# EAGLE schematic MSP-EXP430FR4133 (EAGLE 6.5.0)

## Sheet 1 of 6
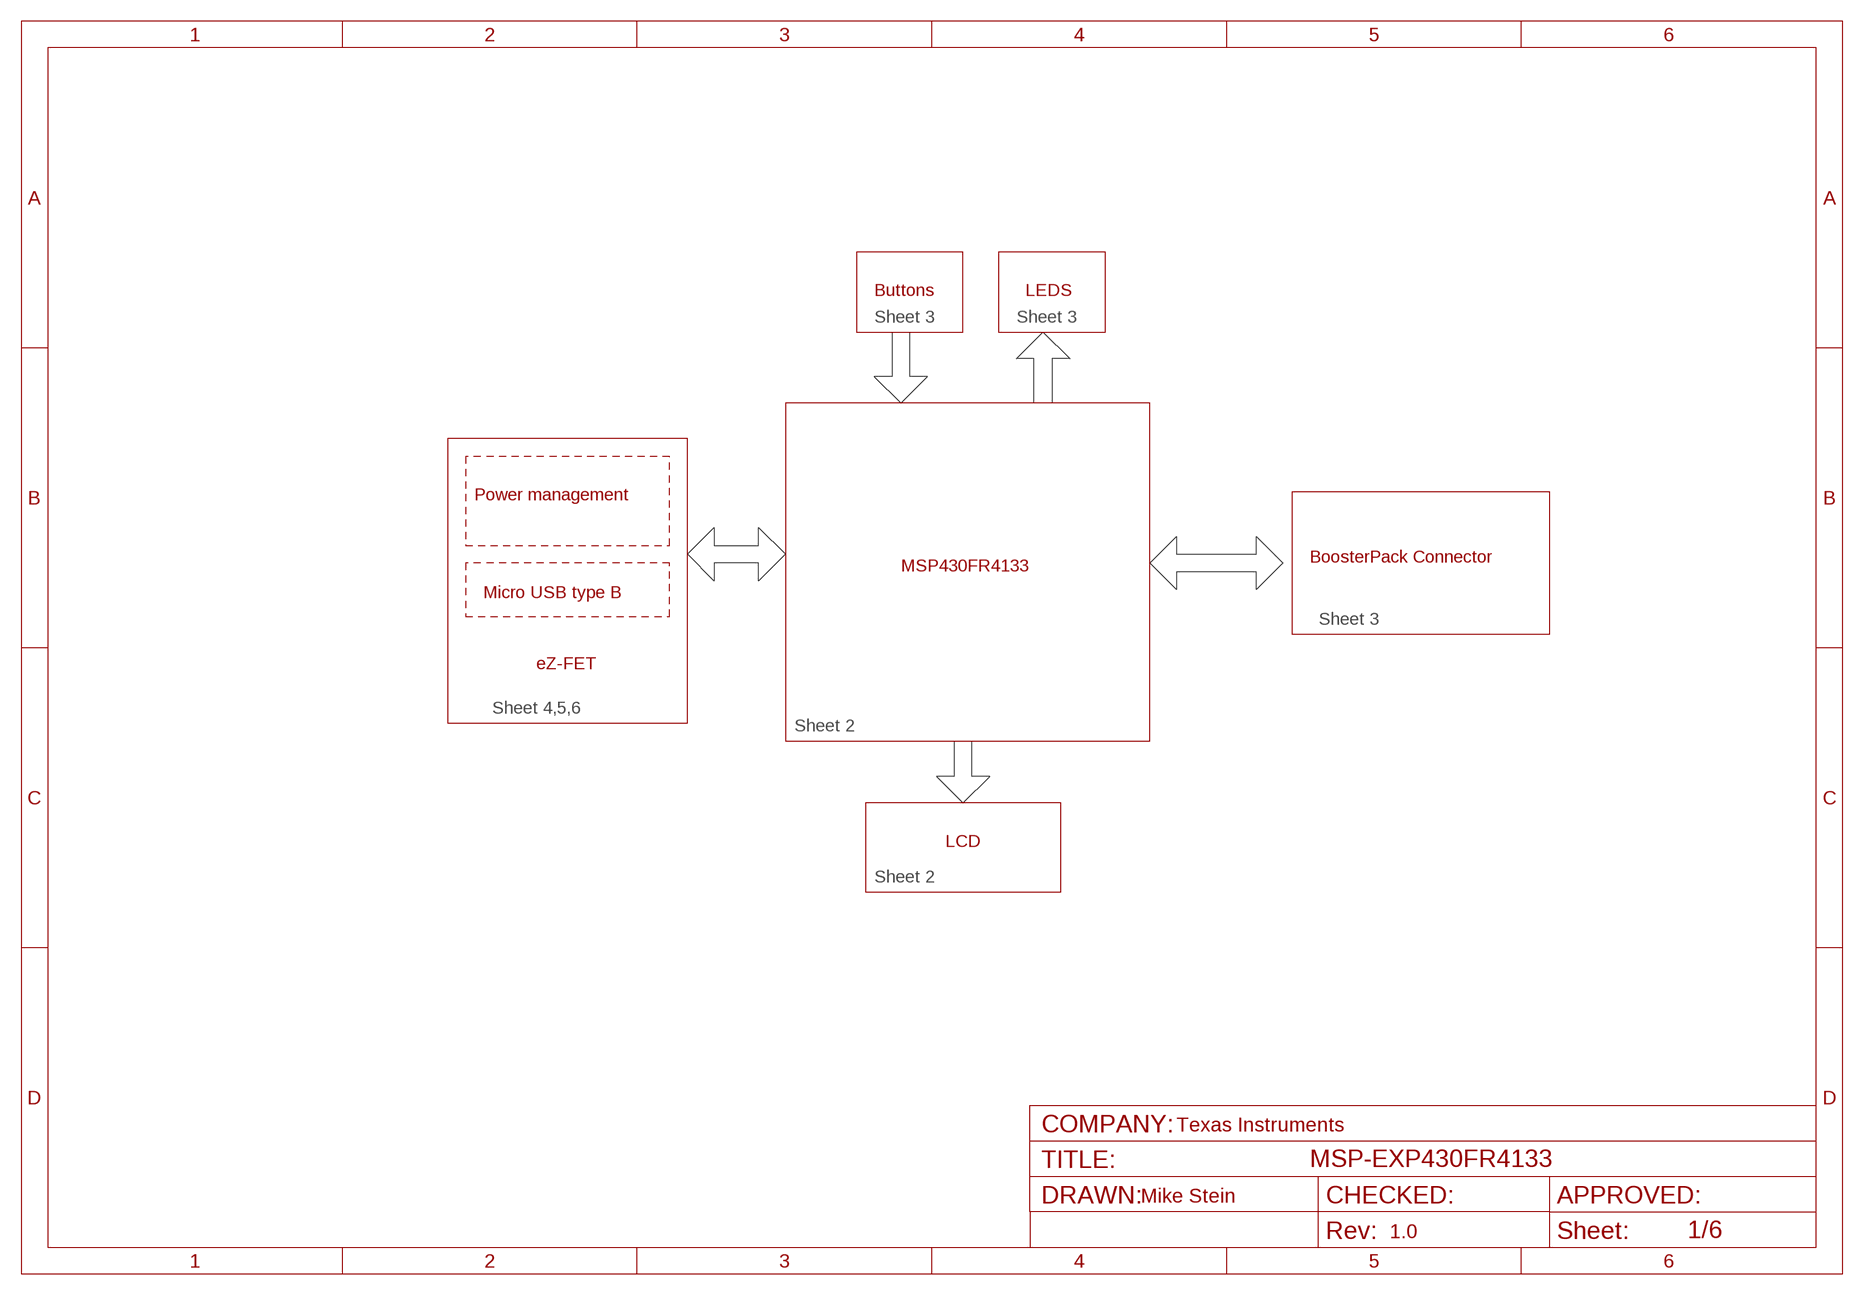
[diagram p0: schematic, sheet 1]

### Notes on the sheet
- Buttons | LEDS
- Sheet 3 | Sheet 3
- Power management
- BoosterPack Connector
- MSP430FR4133
- Micro USB type B
- Sheet 3
- eZ-FET
- Sheet 4,5,6
- Sheet 2
- LCD
- Sheet 2
- Texas Instruments
- Mike Stein
- 1.0

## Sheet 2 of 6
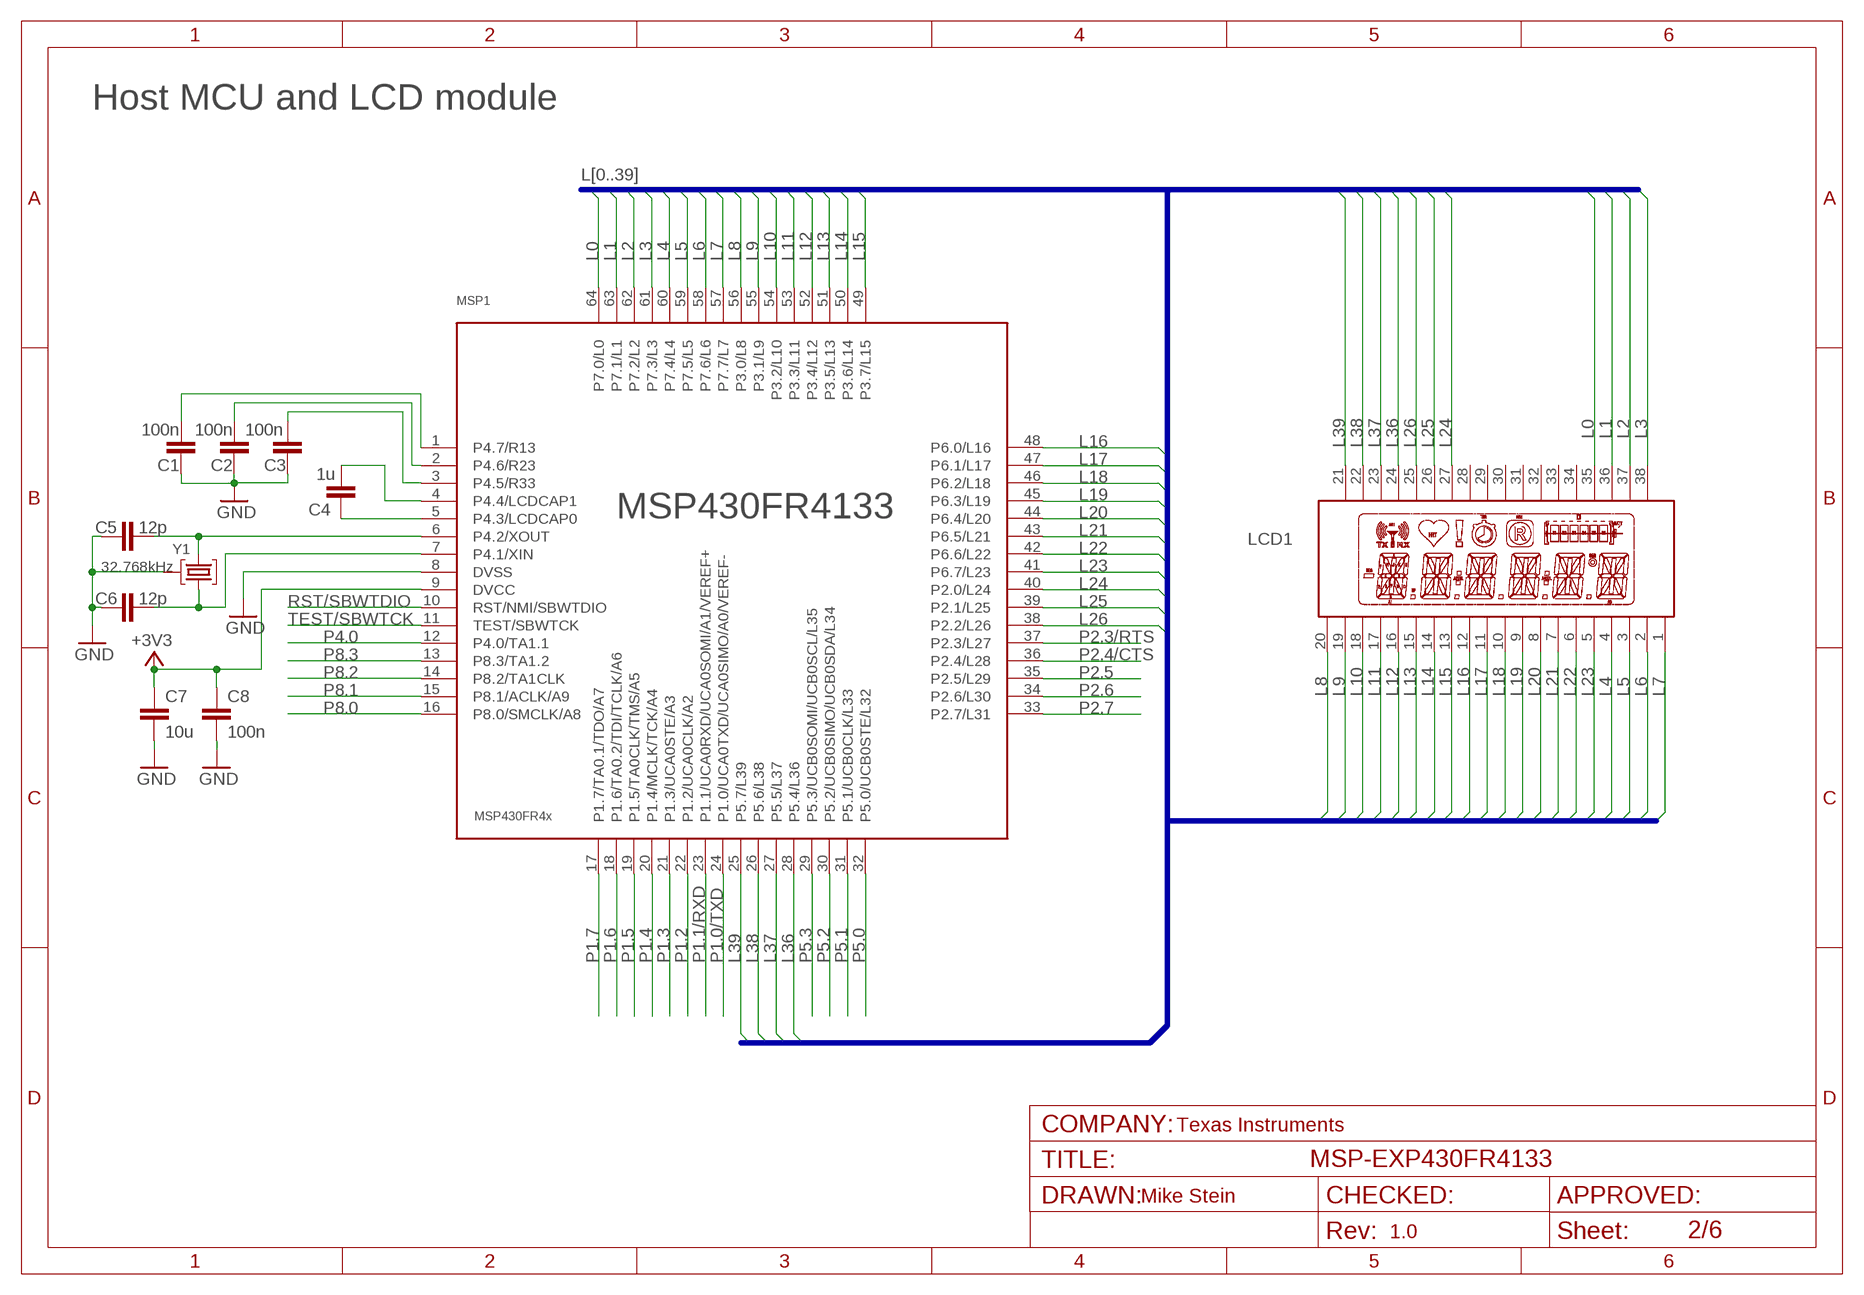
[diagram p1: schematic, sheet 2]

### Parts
C1  100n  C-EUC0402  [C0402]
C2  100n  C-EUC0402  [C0402]
C3  100n  C-EUC0402  [C0402]
C4  1u  C-EUC0402  [C0402]
C5  12p  C-EUC0402  [C0402]
C6  12p  C-EUC0402  [C0402]
C7  10u  C-EUC0603  [C0603]
C8  100n  C-EUC0402  [C0402]
LCD1  FH1138P  [FH1138P]
MSP1  MSP430FR4x  MSP430G621IPM  [LQFP64]
Y1  32.768kHz  MS3V-T1R  [MS3V-T1R]

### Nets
+3V3: C7.1 C8.1 MSP1.9(DVCC) ; also sheet 3,5
GND: C1.2 C2.2 C3.2 C5.2 C6.2 C7.2 C8.2 MSP1.8(DVSS) Y1.P3(GND) ; also sheet 3,4,5,6
L0: LCD1.35 MSP1.64(P7.0/L0)
L1: LCD1.36 MSP1.63(P7.1/L1)
L2: LCD1.37 MSP1.62(P7.2/L2)
L3: LCD1.38 MSP1.61(P7.3/L3)
L4: LCD1.4 MSP1.60(P7.4/L4)
L5: LCD1.3 MSP1.59(P7.5/L5)
L6: LCD1.2 MSP1.58(P7.6/L6)
L7: LCD1.1 MSP1.57(P7.7/L7)
L8: LCD1.20 MSP1.56(P3.0/L8)
L9: LCD1.19 MSP1.55(P3.1/L9)
L10: LCD1.18 MSP1.54(P3.2/L10)
L11: LCD1.17 MSP1.53(P3.3/L11)
L12: LCD1.16 MSP1.52(P3.4/L12)
L13: LCD1.15 MSP1.51(P3.5/L13)
L14: LCD1.14 MSP1.50(P3.6/L14)
L15: LCD1.13 MSP1.49(P3.7/L15)
L16: LCD1.12 MSP1.48(P6.0/L16)
L17: LCD1.11 MSP1.47(P6.1/L17)
L18: LCD1.10 MSP1.46(P6.2/L18)
L19: LCD1.9 MSP1.45(P6.3/L19)
L20: LCD1.8 MSP1.44(P6.4/L20)
L21: LCD1.7 MSP1.43(P6.5/L21)
L22: LCD1.6 MSP1.42(P6.6/L22)
L23: LCD1.5 MSP1.41(P6.7/L23)
L24: LCD1.27 MSP1.40(P2.0/L24)
L25: LCD1.26 MSP1.39(P2.1/L25)
L26: LCD1.25 MSP1.38(P2.2/L26)
L36: LCD1.24 MSP1.28(P5.4/L36)
L37: LCD1.23 MSP1.27(P5.5/L37)
L38: LCD1.22 MSP1.26(P5.6/L38)
L39: LCD1.21 MSP1.25(P5.7/L39)
N$4: C1.1 MSP1.1(P4.7/R13)
N$10: C2.1 MSP1.2(P4.6/R23)
N$11: C4.1 MSP1.4(P4.4/LCDCAP1)
N$14: C5.1 MSP1.6(P4.2/XOUT) Y1.P2
N$17: C4.2 MSP1.5(P4.3/LCDCAP0)
N$18: C6.1 MSP1.7(P4.1/XIN) Y1.P1
N$19: C3.1 MSP1.3(P4.5/R33)
P1.0/TXD: MSP1.24(P1.0/UCA0TXD/UCA0SIMO/A0/VEREF-) ; also sheet 3,5
P1.1/RXD: MSP1.23(P1.1/UCA0RXD/UCA0SOMI/A1/VEREF+) ; also sheet 3,5
P1.2: MSP1.22(P1.2/UCA0CLK/A2) ; also sheet 3
P1.3: MSP1.21(P1.3/UCA0STE/A3) ; also sheet 3
P1.4: MSP1.20(P1.4/MCLK/TCK/A4) ; also sheet 3
P1.5: MSP1.19(P1.5/TA0CLK/TMS/A5) ; also sheet 3
P1.6: MSP1.18(P1.6/TA0.2/TDI/TCLK/A6) ; also sheet 3
P1.7: MSP1.17(P1.7/TA0.1/TDO/A7) ; also sheet 3
P2.3/RTS: MSP1.37(P2.3/L27) ; also sheet 5
P2.4/CTS: MSP1.36(P2.4/L28) ; also sheet 5
P2.5: MSP1.35(P2.5/L29) ; also sheet 3
P2.6: MSP1.34(P2.6/L30) ; also sheet 3
P2.7: MSP1.33(P2.7/L31) ; also sheet 3
P4.0: MSP1.12(P4.0/TA1.1) ; also sheet 3
P5.0: MSP1.32(P5.0/UCB0STE/L32) ; also sheet 3
P5.1: MSP1.31(P5.1/UCB0CLK/L33) ; also sheet 3
P5.2: MSP1.30(P5.2/UCB0SIMO/UCB0SDA/L34) ; also sheet 3
P5.3: MSP1.29(P5.3/UCB0SOMI/UCB0SCL/L35) ; also sheet 3
P8.0: MSP1.16(P8.0/SMCLK/A8) ; also sheet 3
P8.1: MSP1.15(P8.1/ACLK/A9) ; also sheet 3
P8.2: MSP1.14(P8.2/TA1CLK) ; also sheet 3
P8.3: MSP1.13(P8.3/TA1.2) ; also sheet 3
RST/SBWTDIO: MSP1.10(RST/NMI/SBWTDIO) ; also sheet 3,5
TEST/SBWTCK: MSP1.11(TEST/SBWTCK) ; also sheet 5
Unconnected: LCD1.28 LCD1.29 LCD1.30 LCD1.31 LCD1.32 LCD1.33 LCD1.34

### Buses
L[0..39]

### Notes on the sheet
- Host MCU and LCD module
- MSP430FR4133
- Texas Instruments
- Mike Stein
- 1.0

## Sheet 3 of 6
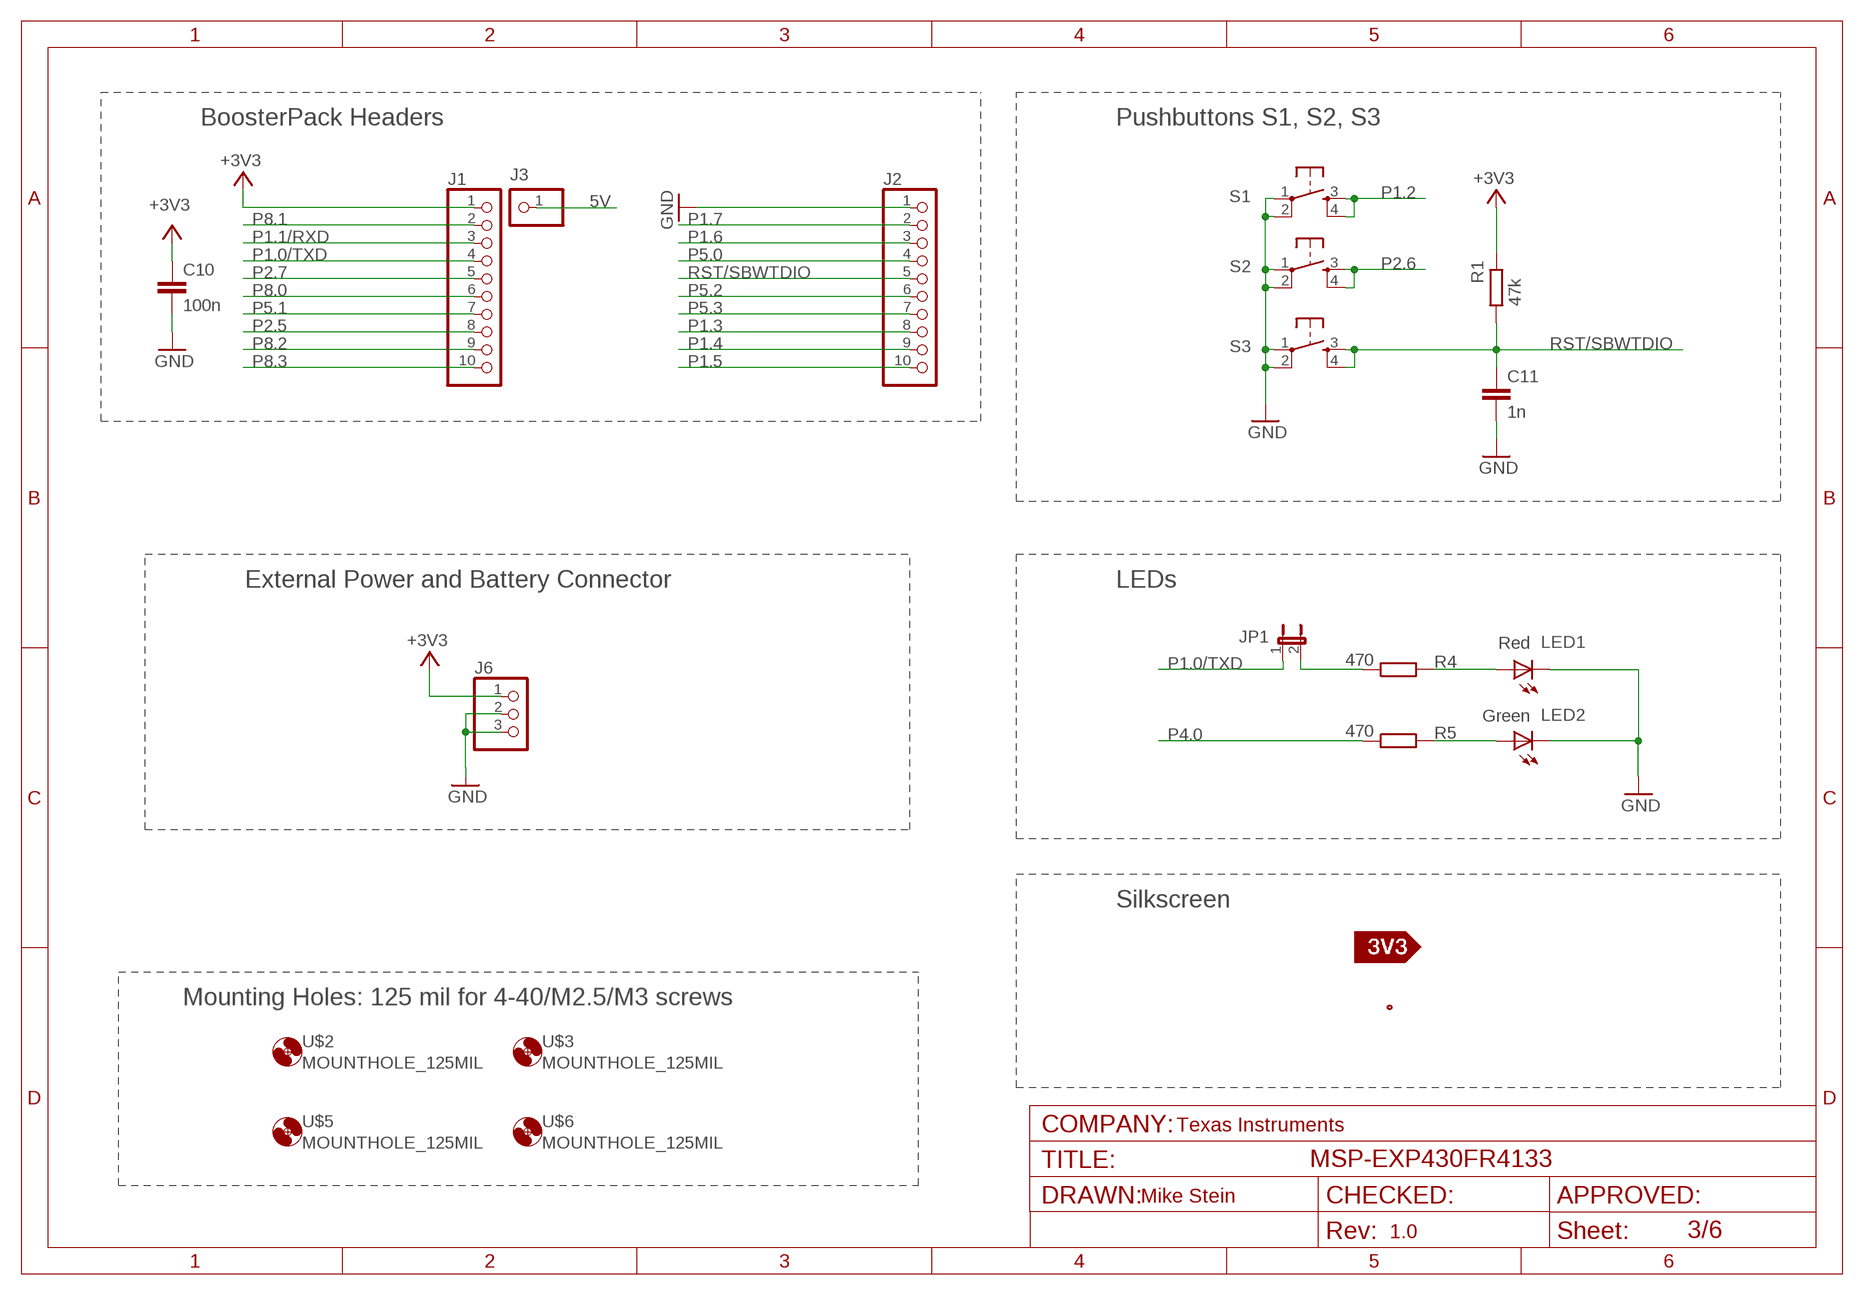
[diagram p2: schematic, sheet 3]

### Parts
C10  100n  C-EUC0402  [C0402]
C11  1n  C-EUC0402  [C0402]
J1  PINHEADER1X10  [PINHEAFER1X10]
J2  PINHEADER1X10  [PINHEAFER1X10]
J3  TEST_PIN2  PINHD-1X1  [1X01]
J6  PINHEADER1X3  [PINHEADER1X3]
JP1  JUMPER_2.51MM  [JUMPER-2.54]
LED1  Red  CHIP-LED  [LED0805]
LED2  Green  CHIP-LED  [LED0805]
R1  47k  R-EU_  [R0402]
R4  470  R-EU_  [R0402]
R5  470  R-EU_  [R0402]
S1  T062S  [T062S]
S2  T062S  [T062S]
S3  T062S  [T062S]
U$2  MOUNTHOLE_125MIL  [MOUNTHOLE_125MIL]
U$3  MOUNTHOLE_125MIL  [MOUNTHOLE_125MIL]
U$5  MOUNTHOLE_125MIL  [MOUNTHOLE_125MIL]
U$6  MOUNTHOLE_125MIL  [MOUNTHOLE_125MIL]
U$7  SILK_3V3_TAG  [SILK_3V3_TAG]
U$8  SILK_FR4133_REAR_REV02  [SILK_FR4133_REAR_REV02]

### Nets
5V: J3.1 ; also sheet 5
+3V3: C10.1 J1.1 J6.1 R1.1 ; also sheet 2,5
GND: C10.2 C11.2 J2.1 J6.2 J6.3 LED1.C LED2.C S1.1 S1.2 S2.1 S2.2 S3.1 S3.2 ; also sheet 2,4,5,6
N$6: JP1.2 R4.1
N$7: LED1.A R4.2
N$8: LED2.A R5.2
P1.0/TXD: J1.4 JP1.1 ; also sheet 2,5
P1.1/RXD: J1.3 ; also sheet 2,5
P1.2: S1.3 S1.4 ; also sheet 2
P1.3: J2.8 ; also sheet 2
P1.4: J2.9 ; also sheet 2
P1.5: J2.10 ; also sheet 2
P1.6: J2.3 ; also sheet 2
P1.7: J2.2 ; also sheet 2
P2.5: J1.8 ; also sheet 2
P2.6: S2.3 S2.4 ; also sheet 2
P2.7: J1.5 ; also sheet 2
P4.0: R5.1 ; also sheet 2
P5.0: J2.4 ; also sheet 2
P5.1: J1.7 ; also sheet 2
P5.2: J2.6 ; also sheet 2
P5.3: J2.7 ; also sheet 2
P8.0: J1.6 ; also sheet 2
P8.1: J1.2 ; also sheet 2
P8.2: J1.9 ; also sheet 2
P8.3: J1.10 ; also sheet 2
RST/SBWTDIO: C11.1 J2.5 R1.2 S3.3 S3.4 ; also sheet 2,5

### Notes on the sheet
- BoosterPack Headers | Pushbuttons S1, S2, S3
- External Power and Battery Connector | LEDs
- Silkscreen
- Mounting Holes: 125 mil for 4-40/M2.5/M3 screws
- Texas Instruments
- Mike Stein
- 1.0

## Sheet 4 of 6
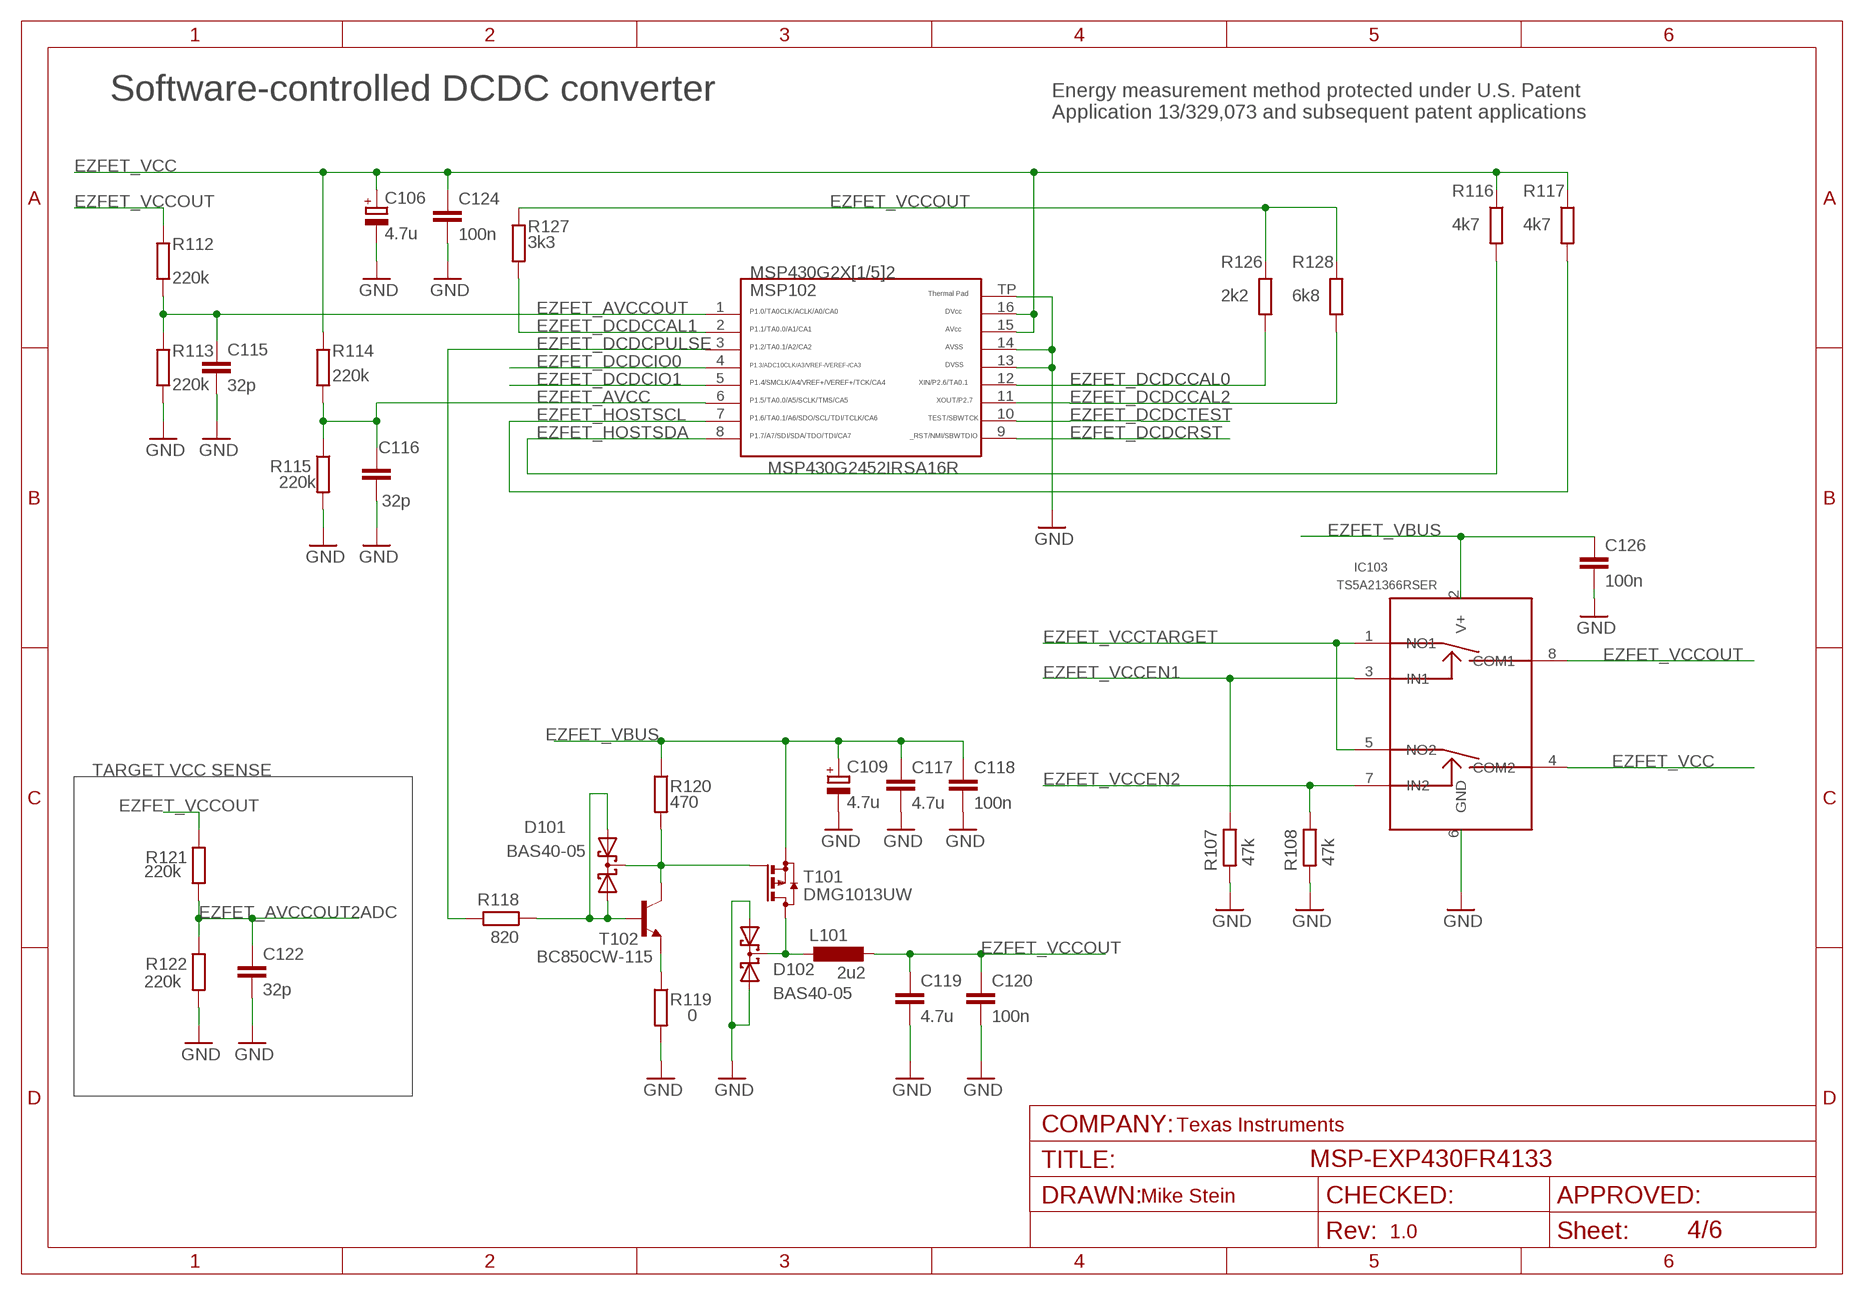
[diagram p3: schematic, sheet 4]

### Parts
C106  4.7u  CPOL-EUA/3216-18R  [A/3216-18R]
C109  4.7u  CPOL-EUA/3216-18R  [A/3216-18R]
C115  32p  C-EUC0402  [C0402]
C116  32p  C-EUC0402  [C0402]
C117  4.7u  C-EUC0603  [C0603]
C118  100n  C-EUC0402  [C0402]
C119  4.7u  C-EUC0603  [C0603]
C120  100n  C-EUC0402  [C0402]
C122  32p  C-EUC0402  [C0402]
C124  100n  C-EUC0402  [C0402]
C126  100n  C-EUC0402  [C0402]
D101  BAS40-05  BAS40-05W  [SOT323]
D102  BAS40-05  BAS40-05W  [SOT323]
IC103  TS5A21366RSER  [UQFN_RSE]
L101  2u2  L-EUL3216C  [L3216C]
MSP102  MSP430G2452IRSA16R  G2X[1/5]2---RSA16  [RSA16]
R107  47k  R-EU_  [R0402]
R108  47k  R-EU_  [R0402]
R112  220k  R-EU_  [R0402]
R113  220k  R-EU_  [R0402]
R114  220k  R-EU_  [R0402]
R115  220k  R-EU_  [R0402]
R116  4k7  R-EU_  [R0402]
R117  4k7  R-EU_  [R0402]
R118  820  R-EU_  [R0402]
R119  0  R-EU_  [R0402]
R120  470  R-EU_  [R0402]
R121  220k  R-EU_  [R0402]
R122  220k  R-EU_  [R0402]
R126  2k2  R-EU_  [R0402]
R127  3k3  R-EU_  [R0402]
R128  6k8  R-EU_  [R0402]
T101  DMG1013UW  [SOT323]
T102  BC850CW-115  [SOT323]

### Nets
EZFET_AVCC: C116.2 MSP102.6 R114.2 R115.1
EZFET_AVCCOUT: C115.2 MSP102.1 R112.2 R113.1
EZFET_AVCCOUT2ADC: C122.2 R121.2 R122.1 ; also sheet 5
EZFET_DCDCCAL0: MSP102.12 R126.2
EZFET_DCDCCAL1: MSP102.2 R127.2
EZFET_DCDCCAL2: MSP102.11 R128.2
EZFET_DCDCIO0: MSP102.4 ; also sheet 5
EZFET_DCDCIO1: MSP102.5 ; also sheet 5
EZFET_DCDCPULSE: MSP102.3 R118.2 ; also sheet 5
EZFET_DCDCRST: MSP102.9 ; also sheet 5,6
EZFET_DCDCTEST: MSP102.10 ; also sheet 5,6
EZFET_HOSTSCL: MSP102.7 R117.2 ; also sheet 5
EZFET_HOSTSDA: MSP102.8 R116.2 ; also sheet 5
EZFET_VBUS: C109.+ C117.1 C118.1 C126.1 IC103.2(V+) R120.1 T101.2(S) ; also sheet 5,6
EZFET_VCC: C106.+ C124.1 IC103.4(COM2) MSP102.15 MSP102.16 R114.1 R116.1 R117.1 ; also sheet 5,6
EZFET_VCCEN1: IC103.3(IN1) R107.1 ; also sheet 5
EZFET_VCCEN2: IC103.7(IN2) R108.1 ; also sheet 5
EZFET_VCCOUT: C119.1 C120.1 IC103.8(COM1) L101.2 R112.1 R121.1 R126.1 R127.1 R128.1
EZFET_VCCTARGET: IC103.1(NO1) IC103.5(NO2) ; also sheet 5
GND: C106.- C109.- C115.1 C116.1 C117.2 C118.2 C119.2 C120.2 C122.1 C124.2 C126.2 D102.1(A1) D102.2(A2) IC103.6(GND) MSP102.13 MSP102.14 MSP102.TP R107.2 R108.2 R113.2 R115.2 R119.2 R122.2 ; also sheet 2,3,5,6
N$12: R119.1 T102.2(E)
N$13: D101.1(A1) D101.2(A2) R118.1 T102.1(B)
N$15: D102.3(C) L101.1 T101.3(D)
N$16: D101.3(C) R120.2 T101.1(G) T102.3(C)

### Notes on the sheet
- Software-controlled DCDC converter
- Energy measurement method protected under U.S. Patent 
  Application 13/329,073 and subsequent patent applications
- MSP430G2452IRSA16R
- TARGET VCC SENSE
- Texas Instruments
- Mike Stein
- 1.0

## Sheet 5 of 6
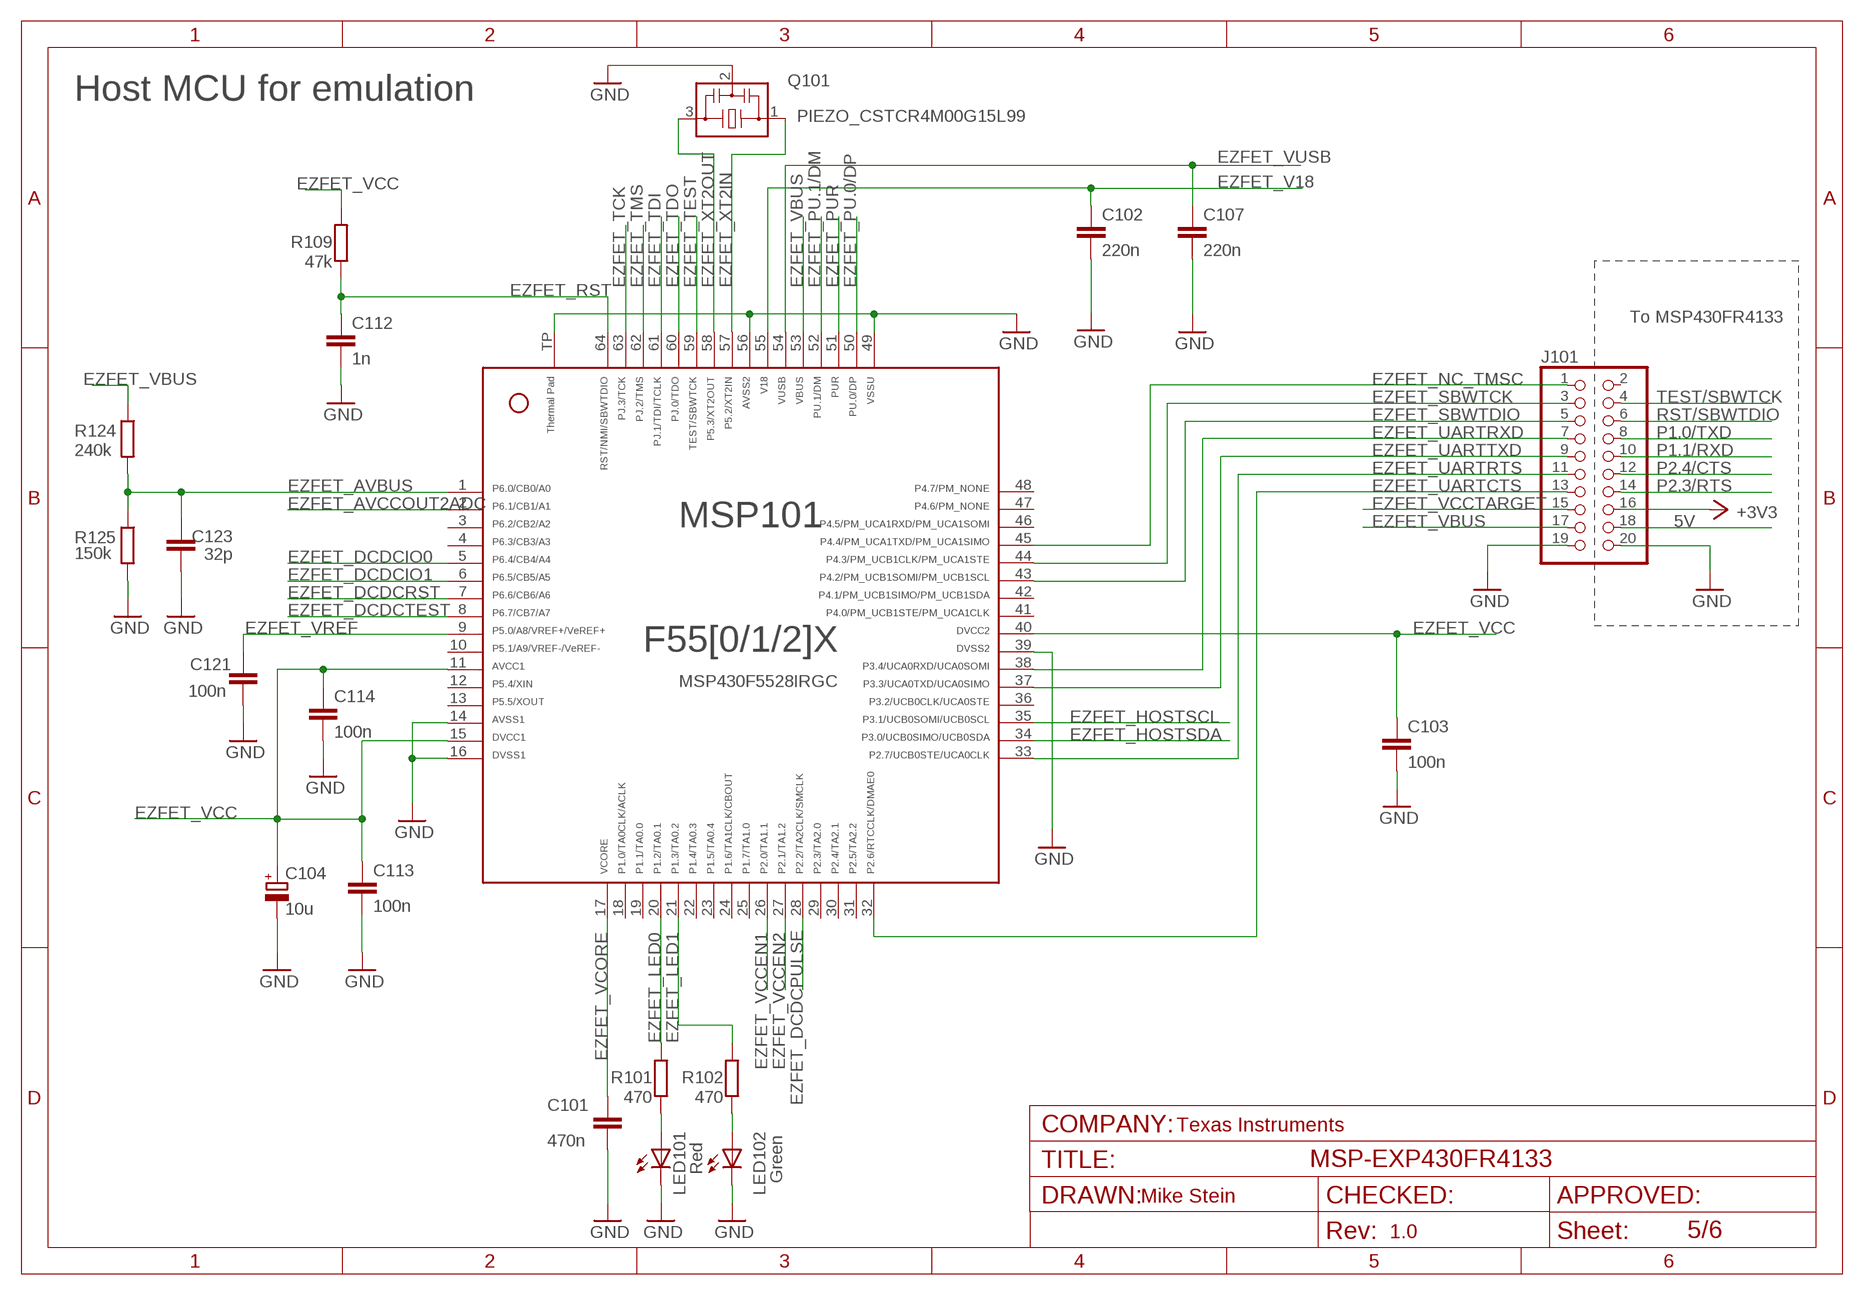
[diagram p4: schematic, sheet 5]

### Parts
C101  470n  C-EUC0402  [C0402]
C102  220n  C-EUC0402  [C0402]
C103  100n  C-EUC0402  [C0402]
C104  10u  CPOL-EUA/3216-18R  [A/3216-18R]
C107  220n  C-EUC0402  [C0402]
C112  1n  C-EUC0402  [C0402]
C113  100n  C-EUC0402  [C0402]
C114  100n  C-EUC0402  [C0402]
C121  100n  C-EUC0402  [C0402]
C123  32p  C-EUC0402  [C0402]
J101  PINHD-2X10  [2X10]
LED101  Red  CHIP-LED  [LED0805]
LED102  Green  CHIP-LED  [LED0805]
MSP101  MSP430F5528IRGC  F55[0/1/2]X---RGC64  [RGC64]
Q101  PIEZO_CSTCR4M00G15L99  CSTCR4M  [CSTCR4M]
R101  470  R-EU_  [R0402]
R102  470  R-EU_  [R0402]
R109  47k  R-EU_  [R0402]
R124  240k  R-EU_  [R0402]
R125  150k  R-EU_  [R0402]

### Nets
5V: J101.18 ; also sheet 3
+3V3: J101.16 ; also sheet 2,3
EZFET_AVBUS: C123.2 MSP101.1 R124.2 R125.1
EZFET_AVCCOUT2ADC: MSP101.2 ; also sheet 4
EZFET_DCDCIO0: MSP101.5 ; also sheet 4
EZFET_DCDCIO1: MSP101.6 ; also sheet 4
EZFET_DCDCPULSE: MSP101.28 ; also sheet 4
EZFET_DCDCRST: MSP101.7 ; also sheet 4,6
EZFET_DCDCTEST: MSP101.8 ; also sheet 4,6
EZFET_HOSTSCL: MSP101.35 ; also sheet 4
EZFET_HOSTSDA: MSP101.34 ; also sheet 4
EZFET_LED0: MSP101.20 R101.2
EZFET_LED1: MSP101.21 R102.2
EZFET_NC_TMSC: J101.1 MSP101.45
EZFET_PU.0/DP: MSP101.50 ; also sheet 6
EZFET_PU.1/DM: MSP101.52 ; also sheet 6
EZFET_PUR: MSP101.51 ; also sheet 6
EZFET_RST: C112.1 MSP101.64 R109.1 ; also sheet 6
EZFET_SBWTCK: J101.3 MSP101.44
EZFET_SBWTDIO: J101.5 MSP101.43
EZFET_TCK: MSP101.63 ; also sheet 6
EZFET_TDI: MSP101.61 ; also sheet 6
EZFET_TDO: MSP101.60 ; also sheet 6
EZFET_TEST: MSP101.59 ; also sheet 6
EZFET_TMS: MSP101.62 ; also sheet 6
EZFET_UARTCTS: J101.13 MSP101.32
EZFET_UARTRTS: J101.11 MSP101.33
EZFET_UARTRXD: J101.7 MSP101.38
EZFET_UARTTXD: J101.9 MSP101.37
EZFET_V18: C102.1 MSP101.55
EZFET_VBUS: J101.17 MSP101.53 R124.1 ; also sheet 4,6
EZFET_VCC: C103.1 C104.+ C113.1 C114.1 MSP101.11 MSP101.15 MSP101.40 R109.2 ; also sheet 4,6
EZFET_VCCEN1: MSP101.26 ; also sheet 4
EZFET_VCCEN2: MSP101.27 ; also sheet 4
EZFET_VCCTARGET: J101.15 ; also sheet 4
EZFET_VCORE: C101.1 MSP101.17
EZFET_VREF: C121.1 MSP101.9
EZFET_VUSB: C107.1 MSP101.54
EZFET_XT2IN: MSP101.57 Q101.1
EZFET_XT2OUT: MSP101.58 Q101.3
GND: C101.2 C102.2 C103.2 C104.- C107.2 C112.2 C113.2 C114.2 C121.2 C123.1 J101.19 J101.20 LED101.C LED102.C MSP101.14 MSP101.16 MSP101.39 MSP101.49 MSP101.56 MSP101.TP Q101.2 R125.2 ; also sheet 2,3,4,6
N$1: LED101.A R101.1
N$2: LED102.A R102.1
P1.0/TXD: J101.8 ; also sheet 2,3
P1.1/RXD: J101.10 ; also sheet 2,3
P2.3/RTS: J101.14 ; also sheet 2
P2.4/CTS: J101.12 ; also sheet 2
RST/SBWTDIO: J101.6 ; also sheet 2,3
TEST/SBWTCK: J101.4 ; also sheet 2
Unconnected: J101.2 MSP101.3 MSP101.4 MSP101.10 MSP101.12 MSP101.13 MSP101.18 MSP101.19 MSP101.22 MSP101.23 MSP101.24 MSP101.25 MSP101.29 MSP101.30 MSP101.31 MSP101.36 MSP101.41 MSP101.42 MSP101.46 MSP101.47 MSP101.48

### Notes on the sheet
- Host MCU for emulation
- To MSP430FR4133
- MSP430F5528IRGC
- Texas Instruments
- Mike Stein
- 1.0

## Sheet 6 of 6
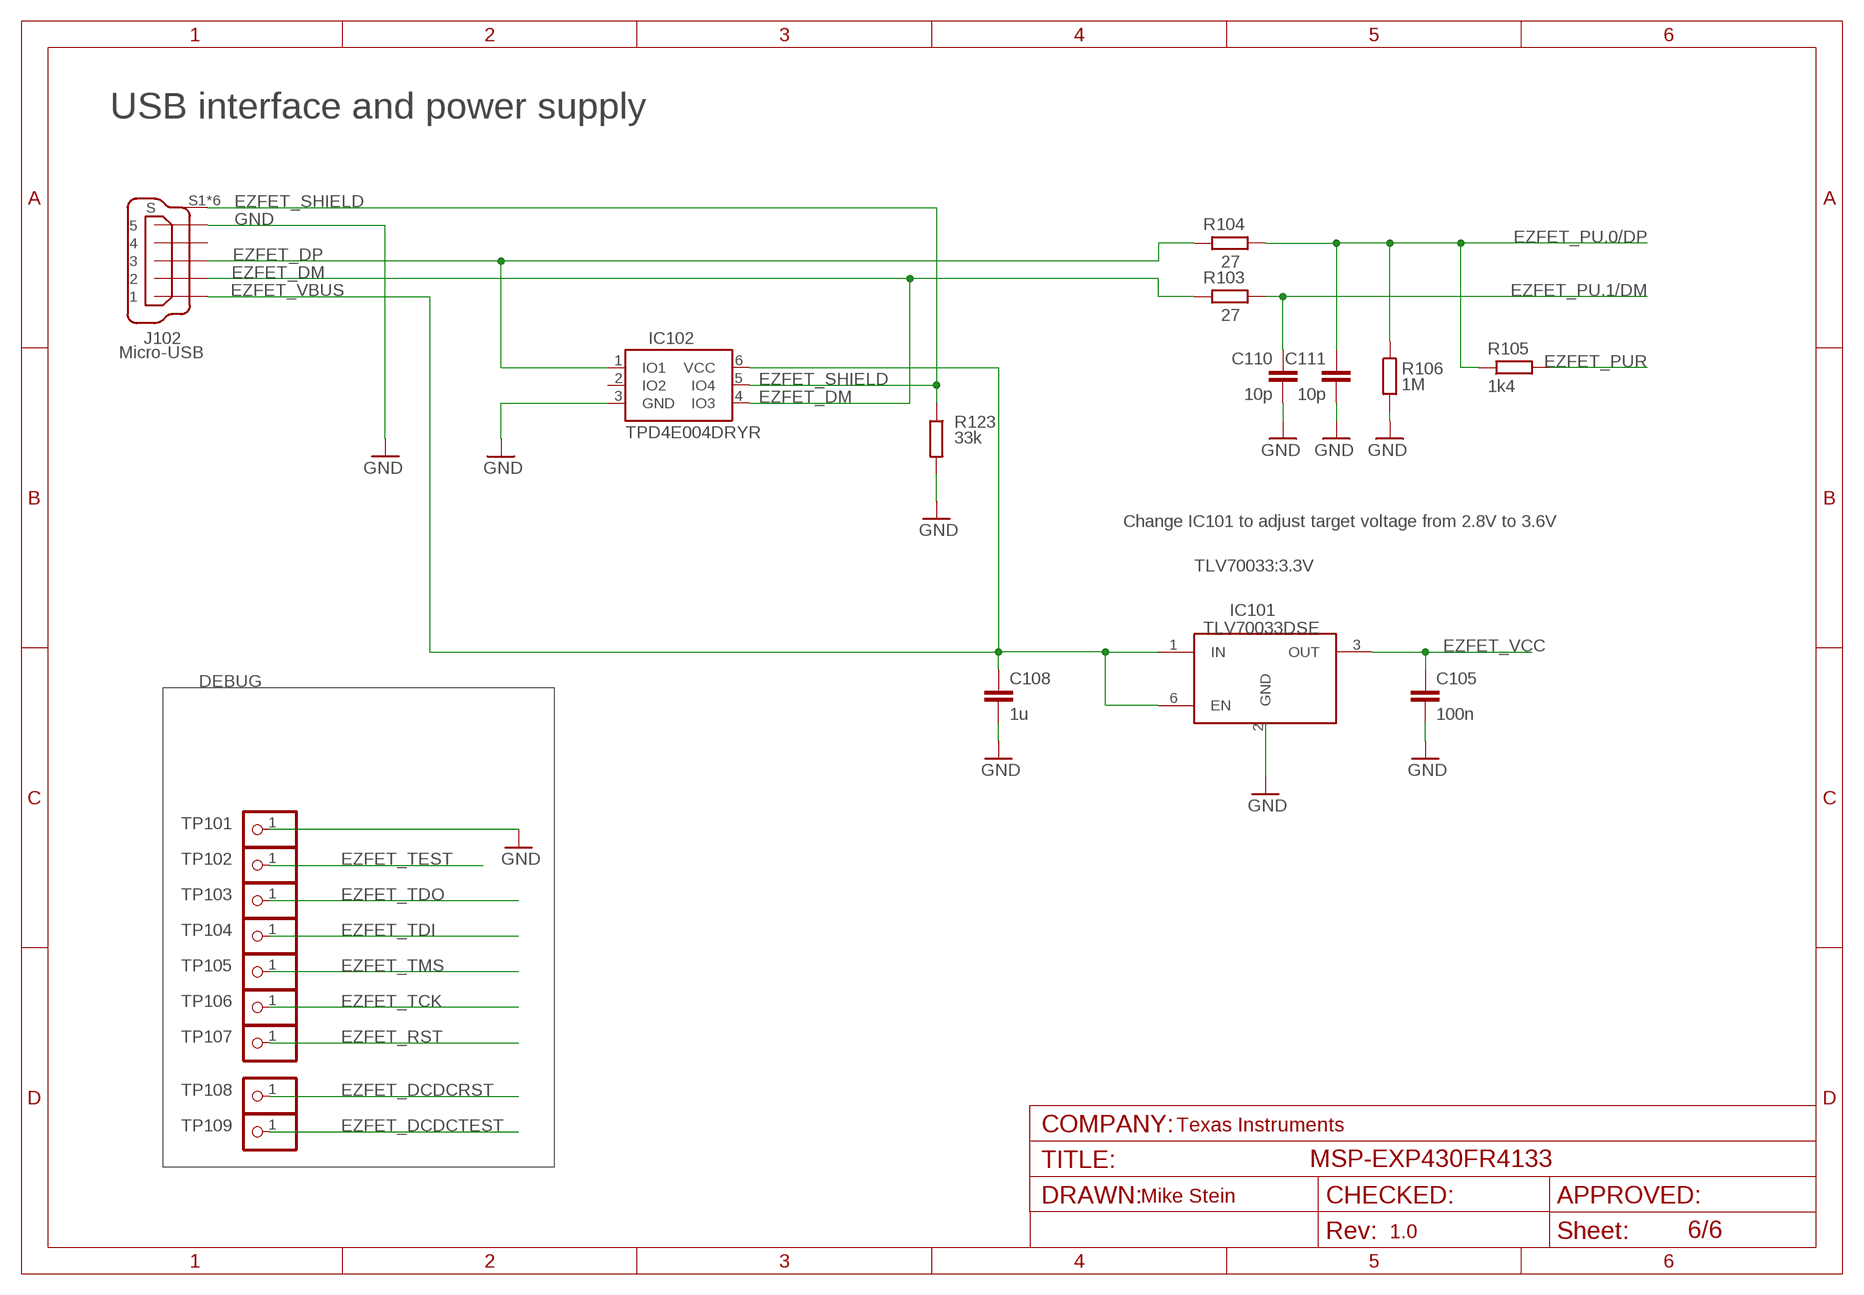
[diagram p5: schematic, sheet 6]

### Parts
C105  100n  C-EUC0402  [C0402]
C108  1u  C-EUC0603  [C0603]
C110  10p  C-EUC0402  [C0402]
C111  10p  C-EUC0402  [C0402]
IC101  TLV70033DSE  [WSON_DSE]
IC102  TPD4E004DRYR  TPD4E004  [SON(DRY)6]
J102  Micro-USB  EZFET_MINI-USB-  [EZFET_UX62M-B-5P]
R103  27  R-EU_  [R0402]
R104  27  R-EU_  [R0402]
R105  1k4  R-EU_  [R0402]
R106  1M  R-EU_  [R0402]
R123  33k  R-EU_  [R0402]
TP101  TEST_PIN2  PINHD-1X1  [1X01]
TP102  TEST_PIN2  PINHD-1X1  [1X01]
TP103  TEST_PIN2  PINHD-1X1  [1X01]
TP104  TEST_PIN2  PINHD-1X1  [1X01]
TP105  TEST_PIN2  PINHD-1X1  [1X01]
TP106  TEST_PIN2  PINHD-1X1  [1X01]
TP107  TEST_PIN2  PINHD-1X1  [1X01]
TP108  TEST_PIN2  PINHD-1X1  [1X01]
TP109  TEST_PIN2  PINHD-1X1  [1X01]

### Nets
EZFET_DCDCRST: TP108.1 ; also sheet 4,5
EZFET_DCDCTEST: TP109.1 ; also sheet 4,5
EZFET_DM: IC102.4(IO3) J102.2 R103.1
EZFET_DP: IC102.1(IO1) J102.3 R104.1
EZFET_PU.0/DP: C111.1 R104.2 R105.1 R106.1 ; also sheet 5
EZFET_PU.1/DM: C110.1 R103.2 ; also sheet 5
EZFET_PUR: R105.2 ; also sheet 5
EZFET_RST: TP107.1 ; also sheet 5
EZFET_SHIELD: IC102.5(IO4) J102.S1(S) J102.S2(S) J102.S3(S) J102.S4(S) J102.S5(S) J102.S6(S) R123.1
EZFET_TCK: TP106.1 ; also sheet 5
EZFET_TDI: TP104.1 ; also sheet 5
EZFET_TDO: TP103.1 ; also sheet 5
EZFET_TEST: TP102.1 ; also sheet 5
EZFET_TMS: TP105.1 ; also sheet 5
EZFET_VBUS: C108.1 IC101.1(IN) IC101.6(EN) IC102.6(VCC) J102.1 ; also sheet 4,5
EZFET_VCC: C105.1 IC101.3(OUT) ; also sheet 4,5
GND: C105.2 C108.2 C110.2 C111.2 IC101.2(GND) IC102.3(GND) J102.5 R106.2 R123.2 TP101.1 ; also sheet 2,3,4,5
Unconnected: IC102.2(IO2) J102.4

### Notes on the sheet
- USB interface and power supply
- Change IC101 to adjust target voltage from 2.8V to 3.6V
- TLV70033:3.3V
- TLV70033DSE
- DEBUG
- Texas Instruments
- Mike Stein
- 1.0

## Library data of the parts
C1-C8 C10 C11 C101-C103 C105 C107 C108 C110-C124 C126 = rcl:C-EU: CAPACITOR, European symbol
C104 C106 C109 = rcl:CPOL-EU: POLARIZED CAPACITOR, European symbol
D101 D102 = MSP430G6_LP:BAS40-05W
IC101 = roy:TLV70033DSE: 200-mA, Low-I Q , Low-Dropout Regulator for Portable Devices
IC102 = eZFET:TPD4E004
IC103 = roy:TS5A21366RSER: 0.75-Ω DUAL SPST ANALOG SWITCH WITH 1.8-V COMPATIBLE INPUT LOGIC
J1 J2 = launchpad:PINHEADER1X10
J3 TP101-TP109 = pinhead:PINHD-1X1: PIN HEADER
J6 = launchpad:PINHEADER1X3
J101 = pinhead:PINHD-2X10: PIN HEADER
J102 = MSP-EXP430G6021:EZFET_MINI-USB-: MINI USB Connector Source: http://www.hirose.co.jp/cataloge_hp/e24000019.pdf
JP1 = launchpad:JUMPER_2.51MM
L101 = rcl:L-EU: INDUCTOR, European symbol
LCD1 = MSP430G6_LP:FH1138P
LED1 LED2 LED101 LED102 = launchpad:CHIP-LED
MSP1 = MSP430G6_LP:MSP430G621IPM
MSP101 = TI_MSP430_v16:F55[0/1/2]X---RGC64: ***F55[0/1/2]X***RGC64 Rev. 1.0 06/2010 "http://www.ti.com/lit/gpn/msp430f5529" "http://www.ti.com/lit/gpn/msp430f5509" F5513/F5514 with limited Functions on some Pins
MSP102 = TI_MSP430_v16:G2X[1/5]2---RSA16: MSP430G2X[1/5]2 MSP430G2x52, MSP430G2x12 QFN (RSA) 16 Pin Package http://focus.ti.com/docs/prod/folders/print/msp430g2452.html
Q101 = MSP430G6_LP:CSTCR4M
R1 R4 R5 R101-R109 R112-R128 = rcl:R-EU_: RESISTOR, European symbol
S1-S3 = launchpad:T062S
T101 = MSP430G6_LP:DMG1013UW
T102 = MSP430G6_LP:BC850CW-115
U$2 U$3 U$5 U$6 = MSP-EXP432:MOUNTHOLE_125MIL
U$7 = MSP-EXP432:SILK_3V3_TAG
U$8 = launchpad:SILK_FR4133_REAR_REV02
Y1 = microcrystal:MS3V-T1R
